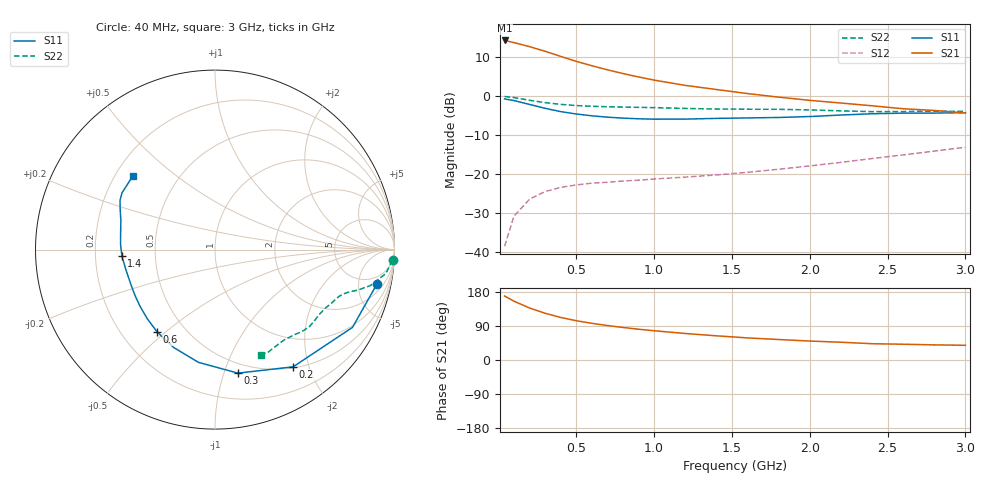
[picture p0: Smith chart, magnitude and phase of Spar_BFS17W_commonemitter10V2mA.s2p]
! Filename:  BFS17WF.S2P  Version:  4.0
! NXP part #: BFS17W  Date: Jun 1994
! Bias condition: Vce=10V, Ic=2mA
#  MHz  S  MA  R  50
! Freq  S11  S21  S12  S22  !GUM [dB]
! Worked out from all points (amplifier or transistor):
!   21 points, 40 MHz to 3 GHz, reference 50 ohm
!   highest |S21| = 14.3 dB at 40 MHz (marker M1)
!   |S21| within 3 dB of that: start of sweep to 317.5 MHz
!   unconditionally stable (mu >= 1): 831.6 MHz to end of sweep
!   at 300 MHz: K = 0.48, MSG = 18.0 dB, |S12| = -24.4 dB
!   at 1 GHz: K = 1.14, MAG = 10.4 dB, |S12| = -21.2 dB
!   at 3 GHz: K = 1.20, MAG = 1.7 dB, |S12| = -13.1 dB
!   S11 on the Smith chart (normalised r, x): 40 MHz: 3.19, -8.22; 200 MHz: 0.52, -1.75; 300 MHz: 0.41, -1.11; 600 MHz: 0.35, -0.47; 1.4 GHz: 0.32, -0.03; 3 GHz: 0.27, +0.36
40  0.922 -12.1  5.177 168.8  0.012 82.0  0.991 -3.4
100  0.88 -29.5  4.86 155.2  0.029 71.3  0.961 -8.0
200  0.785 -56.3  4.315 137.3  0.048 58.6  0.887 -13.1
300  0.7 -79.5  3.763 123.3  0.06 50.7  0.828 -15.8
400  0.635 -98.3  3.237 112.3  0.068 46.7  0.786 -17.4
500  0.592 -112.9  2.795 103.7  0.073 45.1  0.759 -18.9
600  0.561 -125.0  2.458 96.8  0.077 44.9  0.743 -20.2
700  0.539 -134.5  2.178 91.0  0.079 45.6  0.733 -21.4
800  0.524 -142.7  1.952 85.9  0.082 47.1  0.726 -22.5
900  0.514 -150.0  1.765 81.2  0.084 48.6  0.72 -23.6
1000  0.508 -156.4  1.608 77.2  0.087 50.6  0.714 -24.8
1200  0.509 -167.5  1.376 70.0  0.092 55.0  0.697 -27.7
1400  0.52 -176.1  1.219 63.8  0.098 60.2  0.685 -31.5
1600  0.527 176.8  1.081 58.3  0.106 65.1  0.681 -35.7
1800  0.534 169.9  0.973 54.1  0.116 70.4  0.679 -39.1
2000  0.549 162.8  0.885 50.0  0.128 75.2  0.668 -42.6
2200  0.574 157.0  0.818 46.9  0.142 79.2  0.649 -46.9
2400  0.596 152.6  0.754 43.0  0.159 82.4  0.634 -52.5
2600  0.607 148.6  0.691 41.6  0.177 84.6  0.636 -58.2
2800  0.608 143.7  0.657 39.9  0.198 86.5  0.644 -62.7
3000  0.615 137.9  0.609 38.8  0.222 87.9  0.639 -66.3
